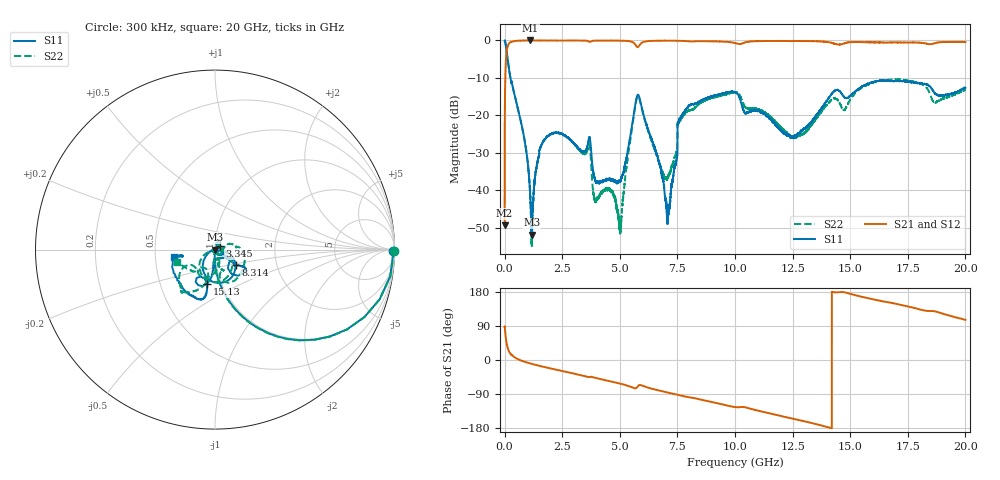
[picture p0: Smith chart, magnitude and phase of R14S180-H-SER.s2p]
!{R14S180}
!Johanson Technology Inc.
!www.johansontechnology.com
!Test Board Conditions:
!Substrate Type  RO4350B
!Substrate Thickness  20 mil
!Substrate Dk  3.66
!TL Type: GCPW
!TL Trace Width  36 mil
!TL Gap  12 mil
!Electrode orientation  Horizontal
!DUT TOPOLOGY	SERIES
!Mounting Pad LxW  26x36 mil
! Created Wed Nov 25 17:33:21 2020
! 2 Port Network Data from SP1.SP block
! freq  magS11  angS11  magS21  angS21  magS12  angS12  magS22  angS22
# khz S ma R 50
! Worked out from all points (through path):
!   20001 points, 300 kHz to 20 GHz, reference 50 ohm
!   highest |S21| = 0.00 dB at 1.112 GHz (marker M1); lowest = -49.3 dB at 300 kHz (marker M2)
!   group delay of S21, straight-line fit = 35.8 ps
!   lowest |S11| = -51.9 dB at 1.182 GHz (marker M3), VSWR 1.01, Z = 50.3 + j0.0393 ohm
!   |S11| at or under -10 dB: 253 MHz to end of sweep
!   |S22| runs from -54.9 to 0.0 dB; largest |S21 - S12| = 0.018
!   S11 on the Smith chart (normalised r, x): 300 kHz: open; 3.345 GHz: 1.05, +0.04; 8.314 GHz: 1.24, -0.22; 15.13 GHz: 0.85, -0.34; 20 GHz: 0.62, -0.05
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300  0.9941 -0.5  0.003416 87.9  0.003342 90.5  0.9987 -0.4
102300  0.6507 -50.2  0.757 39.8  0.7576 39.7  0.6519 -50.2
154300  0.4892 -61.8  0.8682 28.1  0.8698 27.9  0.4919 -61.8
890300  0.04207 -91.9  0.9976 -5.1  0.9978 -5.0  0.04252 -97.1
1112300  0.008521 -82.2  0.9999 -9.1  0.9983 -9.1  0.008778 -111.9
1182300  0.002536 8.9  0.9985 -10.3  0.9989 -10.3  0.001789 155.7
1783300  0.04943 69.8  0.9975 -19.3  0.9976 -19.3  0.04907 70.6
3334300  0.03312 39.8  0.9962 -40.2  0.9966 -40.3  0.03189 49.4
3345300  0.03283 39.0  0.9961 -40.4  0.9955 -40.4  0.03176 49.6
3935300  0.01351 -69.2  0.9936 -47.1  0.994 -47.2  0.007045 -152.8
4988300  0.01289 -52.6  0.9932 -62.0  0.9933 -62.0  0.003353 111.0
5765300  0.1862 -66.6  0.8147 -71.1  0.8151 -71.1  0.1781 -77.5
6667300  0.02594 -158.8  0.9909 -80.0  0.9906 -80.0  0.02512 -152.3
7105300  0.004861 86.4  0.9929 -86.2  0.9927 -86.2  0.01553 -81.8
7600300  0.08973 -35.7  0.9873 -93.1  0.9878 -93.0  0.0845 22.4
8314300  0.1437 -37.2  0.9774 -101.8  0.9757 -101.7  0.1298 6.1
1.00003e7  0.204 -41.7  0.9234 -124.3  0.9234 -124.3  0.2043 -57.7
1.23493e7  0.0538 -69.6  0.9806 -152.6  0.9838 -152.6  0.0543 -74.4
1.33343e7  0.08183 -95.6  0.9802 -166.4  0.981 -166.4  0.07454 -71.3
1.51283e7  0.1976 -102.7  0.9506 172.5  0.9532 172.3  0.1843 -105.4
1.66673e7  0.2886 -112.9  0.9402 152.2  0.9323 152.0  0.2989 -127.2
2e7  0.234 -170.2  0.9516 106.0  0.952 106.1  0.2199 -162.0
